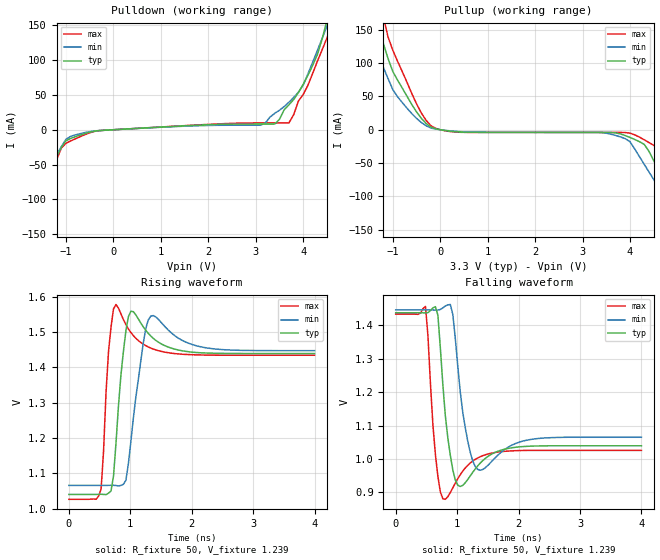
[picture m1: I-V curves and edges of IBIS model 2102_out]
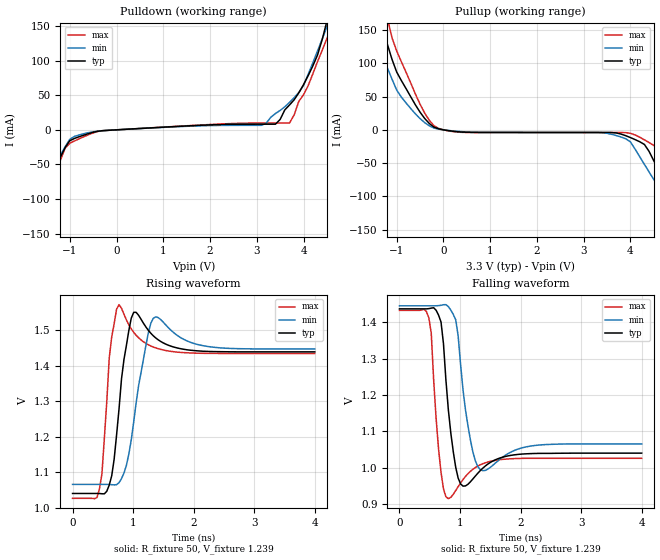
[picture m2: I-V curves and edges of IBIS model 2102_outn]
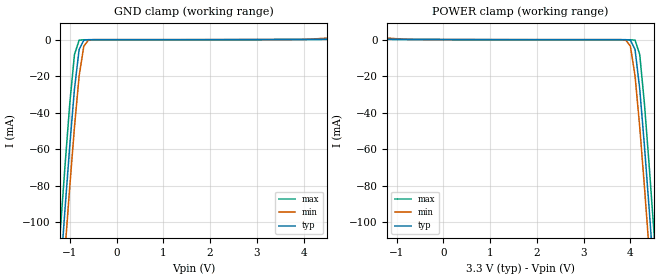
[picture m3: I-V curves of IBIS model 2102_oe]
| IBIS File eg2102l1.ibs
[IBIS ver]   3.2
[File name]   eg2102l1.ibs
[File Rev]   5
[Date]   June 23,2011
[Source]   Circiuts Simulation for EG-2102CA LVDS by HSPICE
|   Component EG-2102CA LVDS
[Component]   EG-2102L
|   (53.125M<=f<=175M)
[Manufacturer]   Epson Toyocom Corp.
[Package]
| variable   typ   min   max
R_pkg   1.04   NA   NA
L_pkg   1.98nH  NA   NA
C_pkg   3.71pF  NA   NA
[Pin]   signal_name   model_name   R_pin   L_pin   C_pin
1   oe   2102_oe   NA   NA   NA
4   out   2102_out   1.04   1.98n   3.71p
5   outn   2102_outn   1.04   1.98n   3.71p
6   vdd   POWER   NA   NA   NA
3   vss   GND   NA   NA   NA
[Diff Pin] inv_pin vdiff   tdelay_typ
4   5   0   0
| Models and submodels in the file (3): 2102_out (Output), 2102_outn (Output), 2102_oe (Input)
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[Model]   2102_out
Model_type Output
Enable Active-High
Polarity Non-Inverting
Vref=1.239
Vmeas=1.239
Rref=50
Cref=0
C_comp   3.81p   3.81p   3.81p
[Temperature Range] 25   85   -40
[Voltage Range]   3.3   3.0   3.6
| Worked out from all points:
|   slope of the pulldown table from 0 to 0.495 V, typ, clamps not added: 258 ohm
|   slope of the pullup table from 0 to 0.495 V, typ, clamps not added: 136 ohm
|   falling waveform, R_fixture 50, V_fixture 1.239: 20-80 % time 97.7ps typ, 126ps min, 74.3ps max; typ from 1.44 V to 1.04 V
|   rising waveform, R_fixture 50, V_fixture 1.239: 20-80 % time 100ps typ, 157ps min, 69ps max; typ from 1.04 V to 1.44 V
[Pullup]
-3.3V     658.9mA    511.8mA    824.7mA
-1.6V     223mA      162.6mA    292.2mA
-1.3V     152.1mA    110.4mA    199mA
-1.2V     128.9mA    93.29mA    168.5mA
-600mV    37.67mA    24.11mA    54.02mA
-100mV    1.437mA    1.025mA    2.076mA
3.4V      -3.979mA   -4.197mA   -4.076mA
4.1V      -14.65mA   -28.92mA   -7.695mA
4.7V      -73.52mA   -96.93mA   -35.21mA
5.3V      -152.5mA   -162.5mA   -133.4mA
5.5V      -180.2mA   -184mA     -169.1mA
6.6V      -314.5mA   -292.7mA   -351.3mA
[Pulldown]
-3.3V     -327.8mA   -277.8mA   -410.2mA
-2.1V     -182.6mA   -154.6mA   -223.5mA
-1.8V     -135.5mA   -116mA     -163.1mA
-1.1V     -25.55mA   -24.41mA   -26.45mA
-900mV    -12.41mA   -9.475mA   -16.06mA
3.1V      8.148mA    6.519mA    9.768mA
3.4V      8.176mA    23.59mA    9.787mA
3.7V      35.85mA    39.53mA    9.814mA
4V        65.18mA    64.05mA    50.54mA
4.5V      156.7mA    148.7mA    131.7mA
4.6V      183.2mA    166.4mA    149.2mA
6.6V      764.4mA    595.7mA    784.3mA
[Falling Waveform]
R_fixture=50
V_fixture=1.239
V_fixture_min=1.256
V_fixture_max=1.23
0s        1.437V     1.446V     1.433V
484.8ps   1.437V     1.446V     1.456V
686.9ps   1.43V      1.446V     947.8mV
767.7ps   1.222V     1.452V     881.2mV
888.9ps   1.011V     1.462V     899.7mV
969.7ps   937.4mV    1.362V     927.8mV
1.131ns   928.9mV    1.095V     972.9mV
1.333ns   979.1mV    969mV      1.003V
2.141ns   1.038V     1.057V     1.026V
4ns       1.04V      1.065V     1.026V
[Rising Waveform]
R_fixture=50
V_fixture=1.239
V_fixture_min=1.256
V_fixture_max=1.23
0s        1.041V     1.066V     1.027V
525.3ps   1.041V     1.066V     1.056V
646.5ps   1.044V     1.066V     1.445V
767.7ps   1.185V     1.066V     1.578V
848.5ps   1.379V     1.066V     1.551V
969.7ps   1.543V     1.128V     1.509V
1.212ns   1.514V     1.469V     1.465V
1.333ns   1.489V     1.545V     1.454V
2.141ns   1.441V     1.458V     1.435V
4ns       1.439V     1.447V     1.434V
[Ramp]
R_load=50
dV/dt_r   2.390E-1/9.753E-11   NA   NA
dV/dt_f   2.387E-1/9.565E-11   NA   NA
|[End   2102_out
[Model]   2102_outn
Model_type Output
Enable Active-High
Polarity Inverting
Vref=1.239
Vmeas=1.239
Rref=50
Cref=0
C_comp   3.81p   3.81p   3.81p
[Temperature Range] 25   85   -40
[Voltage Range]   3.3   3.0   3.6
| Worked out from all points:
|   slope of the pulldown table from 0 to 0.495 V, typ, clamps not added: 258 ohm
|   slope of the pullup table from 0 to 0.495 V, typ, clamps not added: 136 ohm
|   falling waveform, R_fixture 50, V_fixture 1.239: 20-80 % time 117ps typ, 144ps min, 88.1ps max; typ from 1.44 V to 1.04 V
|   rising waveform, R_fixture 50, V_fixture 1.239: 20-80 % time 134ps typ, 202ps min, 93.1ps max; typ from 1.04 V to 1.44 V
[Pullup]
-3.3V     658.9mA    511.8mA    824.7mA
-1.6V     223mA      162.6mA    292.2mA
-1.3V     152.1mA    110.4mA    199mA
-1.2V     128.9mA    93.29mA    168.5mA
-600mV    37.67mA    24.11mA    54.02mA
-100mV    1.437mA    1.025mA    2.076mA
3.4V      -3.979mA   -4.197mA   -4.076mA
4.1V      -14.65mA   -28.92mA   -7.695mA
4.7V      -73.52mA   -96.93mA   -35.21mA
5.3V      -152.5mA   -162.5mA   -133.4mA
5.5V      -180.2mA   -184mA     -169.1mA
6.6V      -314.5mA   -292.7mA   -351.3mA
[Pulldown]
-3.3V     -327.8mA   -277.8mA   -410.2mA
-2.1V     -182.6mA   -154.6mA   -223.5mA
-1.8V     -135.5mA   -116mA     -163.1mA
-1.1V     -25.55mA   -24.41mA   -26.45mA
-900mV    -12.41mA   -9.475mA   -16.06mA
3.1V      8.148mA    6.519mA    9.768mA
3.4V      8.176mA    23.59mA    9.787mA
3.7V      35.85mA    39.53mA    9.814mA
4V        65.18mA    64.05mA    50.54mA
4.5V      156.7mA    148.7mA    131.7mA
4.6V      183.2mA    166.4mA    149.2mA
6.6V      764.4mA    595.7mA    784.3mA
[Falling Waveform]
R_fixture=50
V_fixture=1.239
V_fixture_min=1.256
V_fixture_max=1.23
0s        1.437V     1.446V     1.433V
484.8ps   1.438V     1.446V     1.413V
525.3ps   1.439V     1.446V     1.371V
686.9ps   1.401V     1.447V     987.3mV
808.1ps   1.159V     1.444V     914.5mV
929.3ps   1.001V     1.408V     936.8mV
1.01ns    955.1mV    1.284V     957.9mV
1.172ns   960.9mV    1.077V     989.7mV
1.333ns   991.5mV    994.8mV    1.008V
4ns       1.04V      1.065V     1.026V
[Rising Waveform]
R_fixture=50
V_fixture=1.239
V_fixture_min=1.256
V_fixture_max=1.23
0s        1.041V     1.066V     1.027V
444.4ps   1.04V      1.066V     1.054V
484.8ps   1.04V      1.066V     1.095V
606.1ps   1.064V     1.066V     1.423V
767.7ps   1.279V     1.071V     1.572V
848.5ps   1.417V     1.098V     1.546V
1.01ns    1.551V     1.242V     1.494V
1.333ns   1.485V     1.534V     1.453V
2.141ns   1.441V     1.457V     1.435V
4ns       1.439V     1.448V     1.435V
[Ramp]
R_load=50
dV/dt_r   2.393E-1/1.303E-10   NA   NA
dV/dt_f   2.385E-1/1.109E-10   NA   NA
|[End   2102_outn
[Model]   2102_oe
Model_type Input
Vinh=2.31
Vinl=0.99
C_comp   3p   3p   3p
[Temperature Range] 25   85   -40
[Voltage Range]   3.3   3.0   3.6
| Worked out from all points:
|   GND clamp passes 1 mA (typ) near -0.71 V on its own axis
|   POWER clamp passes 1 mA (typ) near -1.64 V on its own axis
[GND Clamp]
-3.3V     -919.3mA   -939.8mA   -898.4mA
-1.3V     -163.5mA   -186.1mA   -139.9mA
-1.2V     -127.3mA   -150mA     -103.6mA
-1.1V     -91.92mA   -114.6mA   -68.2mA
-1V       -57.9mA    -80.23mA   -34.85mA
-900mV    -26.97mA   -47.81mA   -8.167mA
-800mV    -5.443mA   -19.86mA   -333.4uA
-700mV    -343.6uA   -3.593mA   -111.9uA
-600mV    -74.3uA    -310.2uA   -110.3uA
4V        43.73uA    87.52uA    33.74uA
4.8V      743.7uA    1.34mA     209.3uA
6.6V      4.189mA    4.806mA    3.578mA
[POWER Clamp]
-3.3V     4.189mA    4.806mA    3.578mA
-1.5V     743.7uA    1.34mA     209.3uA
-700mV    43.73uA    87.52uA    33.74uA
3.9V      -74.3uA    -310.2uA   -110.3uA
4V        -343.6uA   -3.593mA   -111.9uA
4.1V      -5.443mA   -19.86mA   -333.4uA
4.2V      -26.97mA   -47.81mA   -8.167mA
4.3V      -57.9mA    -80.23mA   -34.85mA
4.4V      -91.92mA   -114.6mA   -68.2mA
4.5V      -127.3mA   -150mA     -103.6mA
4.6V      -163.5mA   -186.1mA   -139.9mA
6.6V      -919.3mA   -939.8mA   -898.4mA
